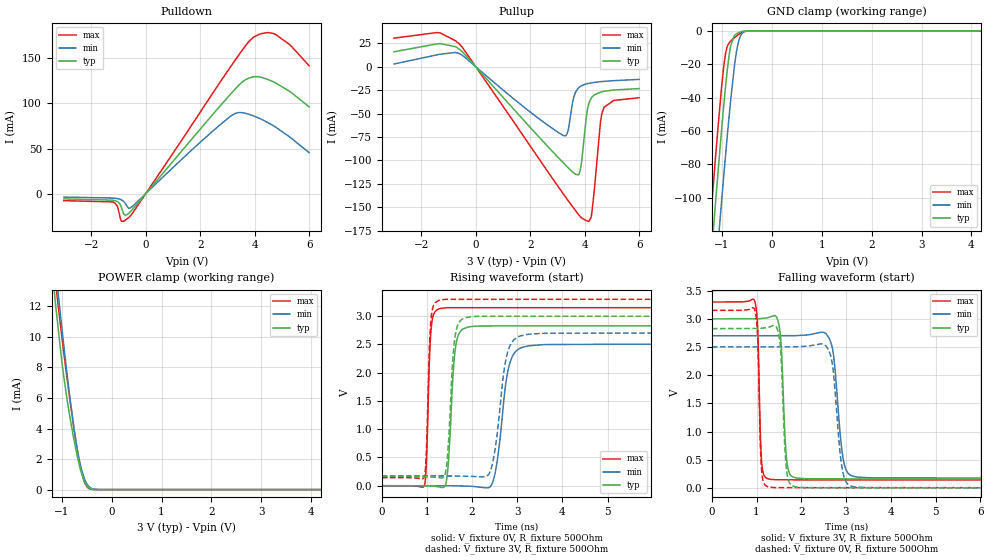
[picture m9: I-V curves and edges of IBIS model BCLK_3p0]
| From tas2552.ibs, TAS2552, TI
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|   Model
[Model]   BCLK_3p0
Model_type   I/O
Polarity   Non-Inverting
Enable   Active-Low
Vinl = 0.9
Vinh = 2.1
Vmeas = 1.5
Vref = 0
Cref = 1pF
Rref = 1000000
|   typ   min   max
C_comp   1.269pF   1.168pF   1.417pF
[Voltage Range]   3   2.7   3.3
[Temperature Range]   27   125   -40
[Pullup Reference]   3   2.7   3.3
[Pulldown Reference]   -0   -0   -0
[Power Clamp Reference]   3   2.7   3.3
[GND Clamp Reference]   -0   -0   -0
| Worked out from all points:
|   slope of the pulldown table from 0 to 0.45 V, typ, clamps not added: 27.9 ohm
|   slope of the pullup table from 0 to 0.45 V, typ, clamps not added: 30.6 ohm
|   GND clamp passes 1 mA (typ) near -0.66 V on its own axis
|   POWER clamp passes 1 mA (typ) near -0.60 V on its own axis
|   falling waveform, V_fixture 3V, R_fixture 500Ohm: 20-80 % time 92.2ps typ, 163ps min, 59.8ps max; typ from 3 V to 0.158 V
|   rising waveform, V_fixture 0V, R_fixture 500Ohm: 20-80 % time 119ps typ, 218ps min, 73ps max; typ from 0 V to 2.83 V
|   rising waveform, V_fixture 3V, R_fixture 500Ohm: 20-80 % time 119ps typ, 224ps min, 72.7ps max; typ from 0.158 V to 3 V
|   falling waveform, V_fixture 0V, R_fixture 500Ohm: 20-80 % time 92.3ps typ, 161ps min, 59.8ps max; typ from 2.83 V to 0 V
[Pulldown]
|   Voltage   I(typ)   I(min)   I(max)
-3V       -5.841mA   -3.822mA   -7.815mA
-1.218V   -7.237mA   -4.925mA   -9.165mA
-1.038V   -8.936mA   -5.569mA   -14.21mA
-894mV    -15mA      -6.834mA   -30.69mA
-750mV    -24.16mA   -10.81mA   -29.53mA
-633mV    -22mA      -15.95mA   -26.79mA
3.129V    110.9mA    86.23mA    141.6mA
3.408V    120.1mA    89.94mA    153.6mA
3.957V    129.7mA    86.19mA    173.6mA
4.479V    126.7mA    78.81mA    178.7mA
4.785V    122.5mA    73.34mA    176.2mA
5.991V    96.26mA    45.47mA    142mA
[GND Clamp]
|   Voltage   I(typ)   I(min)   I(max)
-3V       -847.1mA   -879.1mA   -828.2mA
-1.335V   -182.1mA   -224.6mA   -155.5mA
-1.164V   -116.9mA   -160.2mA   -89.71mA
-1.101V   -93.58mA   -136.9mA   -66.47mA
-1.011V   -61.43mA   -104.4mA   -35.62mA
-930mV    -34.8mA    -76.13mA   -14.5mA
-822mV    -8.814mA   -41.3mA    -6.147mA
-732mV    -2.338mA   -17.61mA   -3.738mA
-660mV    -1.043mA   -5.862mA   -2.126mA
-579mV    -318.1uA   -1.113mA   -788.5uA
-435mV    -12.78uA   -34.01uA   -30.82uA
5.991V    0A         0A         0A
[Pullup]
|   Voltage   I(typ)   I(min)   I(max)
-3V       16.06mA    3.006mA    30.62mA
-1.434V   24.43mA    12.69mA    36.59mA
-606mV    18.86mA    14.15mA    24.44mA
3.237V    -103.4mA   -73.66mA   -136.9mA
3.372V    -107.4mA   -69.34mA   -142.4mA
3.669V    -114.9mA   -26.48mA   -154.2mA
3.831V    -110.4mA   -21.08mA   -160.1mA
4.101V    -44.59mA   -17.94mA   -164.9mA
4.254V    -32.64mA   -17.06mA   -156.4mA
4.569V    -27.08mA   -15.9mA    -60.03mA
4.695V    -26.21mA   -15.57mA   -43.79mA
5.991V    -23.28mA   -13.43mA   -33.03mA
[POWER Clamp]
|   Voltage   I(typ)   I(min)   I(max)
-3V       84.31mA    76.07mA    99.07mA
-1.137V   12.62mA    14.88mA    13.96mA
-1.119V   12.03mA    14.32mA    13.44mA
-1.011V   8.785mA    11.02mA    10.4mA
-894mV    5.939mA    7.615mA    7.321mA
-750mV    3.191mA    3.91mA     3.906mA
-660mV    1.792mA    2.136mA    2.109mA
-579mV    824.7uA    1.044mA    878.9uA
-507mV    291.5uA    447.8uA    253.9uA
-435mV    68.49uA    143.4uA    45.74uA
-174mV    127.6nA    300nA      0A
5.991V    0A         0A         0A
[Ramp]
R_load = 500
|   typ   min   max
dV/dt_r   1.69648/1.18993e-10   1.50106/2.17992e-10   1.89049/7.30361e-11
dV/dt_f   1.70491/9.21953e-11   1.51629/1.63001e-10   1.89533/5.97629e-11
[Falling Waveform]
V_fixture = 3V
V_fixture_min = 2.7V
V_fixture_max = 3.3V
R_fixture = 500Ohm
C_fixture = 0F
|   Time   V(typ)   V(min)   V(max)
0s        3V         2.7V       3.3V
956.9ps   3.001V     2.701V     3.32V
1.119ns   3.008V     2.701V     408.1mV
1.422ns   3.053V     2.702V     144.9mV
1.699ns   352.6mV    2.702V     143.3mV
2.087ns   162.9mV    2.713V     141.8mV
2.62ns    160.6mV    2.661V     141.1mV
2.958ns   159.7mV    428.6mV    141.1mV
3.49ns    158.5mV    179.9mV    141.1mV
100ns     158.5mV    172.8mV    141.1mV
[Rising Waveform]
V_fixture = 0V
V_fixture_min = 0V
V_fixture_max = 0V
R_fixture = 500Ohm
C_fixture = 0F
|   Time   V(typ)   V(min)   V(max)
0s        1.927nV    18.89nV    1.168nV
948.2ps   -628.8uV   3.668uV    15.6mV
1.109ns   -6.851mV   4.287uV    2.886V
1.446ns   166.3mV    5.583uV    3.148V
1.651ns   2.531V     -2.045mV   3.148V
2.126ns   2.823V     -21.12mV   3.148V
2.47ns    2.825V     93.86mV    3.148V
2.873ns   2.826V     2.253V     3.148V
3.568ns   2.827V     2.495V     3.148V
100ns     2.827V     2.502V     3.151V
[Rising Waveform]
V_fixture = 3V
V_fixture_min = 2.7V
V_fixture_max = 3.3V
R_fixture = 500Ohm
C_fixture = 0F
|   Time   V(typ)   V(min)   V(max)
0s        158.5mV    172.8mV    141.1mV
934.7ps   157.6mV    172.5mV    143.4mV
1.099ns   152.7mV    172.4mV    3.004V
1.422ns   277.5mV    172.3mV    3.297V
1.637ns   2.703V     171mV      3.297V
2.126ns   2.996V     160.3mV    3.297V
2.433ns   2.996V     332.9mV    3.297V
2.845ns   2.996V     2.486V     3.297V
3.568ns   2.996V     2.694V     3.297V
100ns     3V         2.7V       3.3V
[Falling Waveform]
|Gnd
V_fixture = 0V
V_fixture_min = 0V
V_fixture_max = 0V
R_fixture = 500Ohm
C_fixture = 0F
|   Time   V(typ)   V(min)   V(max)
0s        2.827V     2.502V     3.151V
956.9ps   2.829V     2.503V     3.166V
1.119ns   2.835V     2.503V     255.3mV
1.422ns   2.874V     2.504V     3.765mV
1.682ns   245.4mV    2.504V     3.755mV
2.048ns   4.657mV    2.512V     3.741mV
2.62ns    2.169mV    2.43V      3.72mV
2.958ns   1.189mV    187.1mV    3.707mV
3.412ns   5.642uV    5.614mV    3.689mV
100ns     13.1nV     30.81nV    9.026nV
